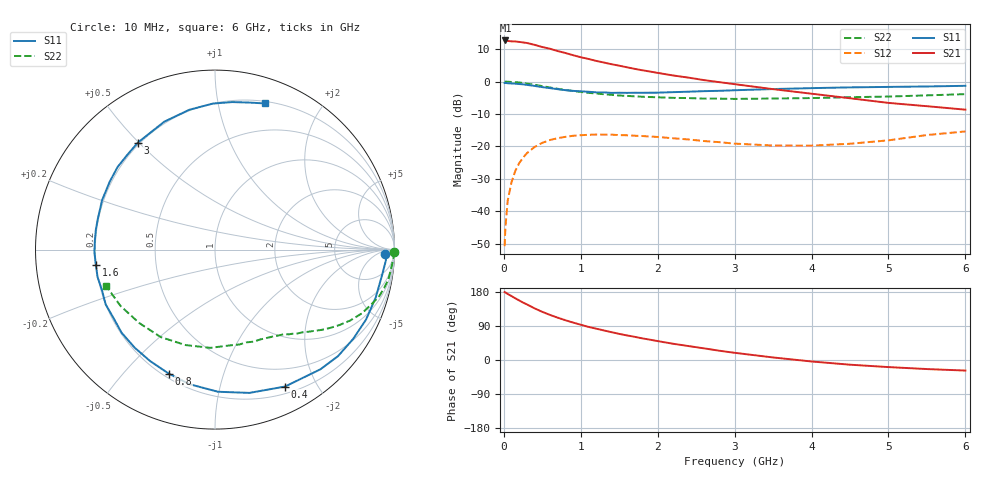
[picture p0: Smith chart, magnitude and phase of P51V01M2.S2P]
! SIEMENS Small Signal Semiconductors
! BFP183
! Si NPN RF Bipolar Junction Transistor in SOT143
! VCE = 1 V  IC = 1.2 mA
! Common Emitter S-Parameters:  March  1996
# GHz  S  MA  R  50
!  f  S11  S21  S12  S22
! GHz  MAG  ANG  MAG  ANG  MAG  ANG  MAG  ANG
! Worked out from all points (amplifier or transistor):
!   36 points, 10 MHz to 6 GHz, reference 50 ohm
!   highest |S21| = 12.7 dB at 20 MHz (marker M1)
!   |S21| within 3 dB of that: start of sweep to 662 MHz
!   unconditionally stable (mu >= 1): 2.328 GHz to end of sweep
!   at 250 MHz: K = 0.11, MSG = 17.8 dB, |S12| = -23.5 dB
!   at 1.4 GHz: K = 0.60, MSG = 10.9 dB, |S12| = -16.4 dB
!   at 6 GHz: K = 1.15, MAG = 1.0 dB, |S12| = -15.4 dB
!   S11 on the Smith chart (normalised r, x): 10 MHz: 31, -16; 400 MHz: 0.28, -1.60; 800 MHz: 0.22, -0.67; 1.6 GHz: 0.20, -0.06; 3 GHz: 0.19, +0.50; 6 GHz: 0.22, +1.37
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0.01  0.9496 -1.5  4.24 179.2  0.0029 87.2  0.9997 -0.7
0.02  0.9544 -3.5  4.304 178.3  0.0055 83.8  0.9993 -1.3
0.05  0.9422 -8.4  4.238 174.3  0.0146 87.4  0.9938 -3.2
0.1  0.9345 -16.5  4.168 168.6  0.0282 79.3  0.9864 -6.5
0.15  0.9275 -24.9  4.154 162.7  0.0423 74.8  0.9798 -9.8
0.25  0.9067 -40.9  4.009 151.5  0.0671 65.8  0.9513 -15.8
0.3  0.8887 -48.6  3.938 146.7  0.0787 61.5  0.9303 -18.4
0.4  0.857 -62.9  3.682 136.2  0.0981 53.2  0.8929 -23.4
0.5  0.8211 -76.5  3.408 127.1  0.1136 45.9  0.8505 -27.7
0.6  0.7922 -88.8  3.205 119.0  0.1256 39.3  0.8099 -31.3
0.8  0.7373 -110.5  2.759 104.9  0.1405 28.5  0.742 -37.1
0.9  0.7186 -120.2  2.551 98.8  0.146 24.2  0.715 -39.3
1.1  0.6967 -138.3  2.235 87.4  0.1511 16.6  0.6709 -43.4
1.3  0.6814 -153.4  1.966 78.0  0.1519 10.2  0.6383 -47.2
1.6  0.6695 -172.6  1.661 64.9  0.1487 3.2  0.6018 -52.1
1.9  0.6731 170.5  1.428 53.6  0.1423 -2.2  0.5776 -57.6
2.2  0.6868 156.3  1.242 42.9  0.1336 -5.2  0.5608 -63.1
3  0.735 125.8  0.912 19.0  0.1105 -6.5  0.5404 -80.5
3.5  0.7668 111.6  0.764 6.7  0.1032 -1.3  0.548 -92.7
4.5  0.8137 90.8  0.553 -12.4  0.11 13.0  0.5737 -121.8
5.5  0.8406 77.1  0.417 -23.9  0.1499 18.9  0.6129 -149.2
6  0.8603 71.2  0.369 -27.9  0.1704 16.4  0.6402 -161.7
